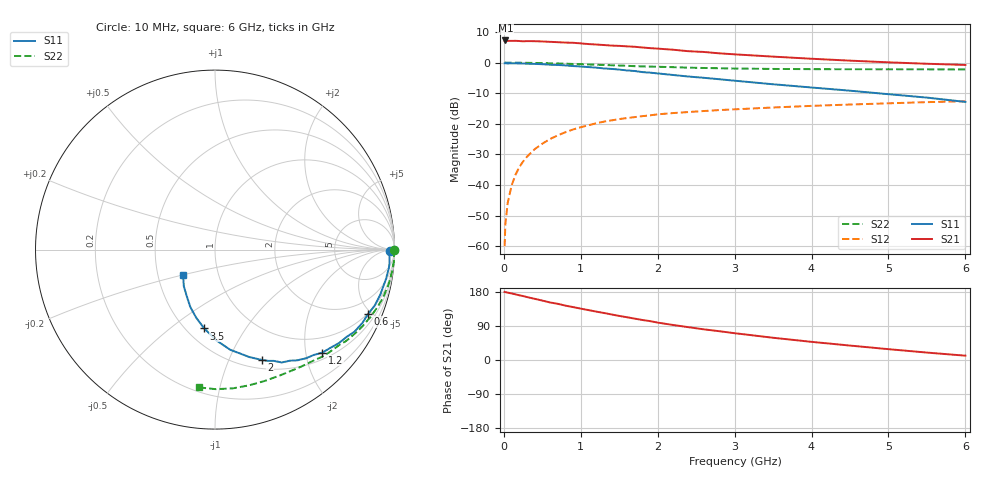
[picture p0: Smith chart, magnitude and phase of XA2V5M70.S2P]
! SIEMENS Discrete & RF Semiconductors
! BFY180
! Si NPN RF Bipolar Junction Transistor in MICRO-X
! VCE = 2.5 V  IC = 0.7 mA
! Common Emitter S-Parameters:  May  1997
# GHz  S  MA  R  50
!  f  S11  S21  S12  S22
! GHz  MAG  ANG  MAG  ANG  MAG  ANG  MAG  ANG
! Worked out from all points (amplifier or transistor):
!   36 points, 10 MHz to 6 GHz, reference 50 ohm
!   highest |S21| = 7.3 dB at 20 MHz (marker M1)
!   |S21| within 3 dB of that: start of sweep to 2.186 GHz
!   unconditionally stable (mu >= 1): 4.433 GHz to end of sweep
!   at 250 MHz: K = 0.07, MSG = 19.6 dB, |S12| = -32.3 dB
!   at 1.4 GHz: K = 0.44, MSG = 12.2 dB, |S12| = -18.9 dB
!   at 6 GHz: K = 1.05, MAG = 4.6 dB, |S12| = -12.6 dB
!   S11 on the Smith chart (normalised r, x): 10 MHz: 73, -14; 600 MHz: 0.96, -4.78; 1.2 GHz: 0.64, -2.34; 2 GHz: 0.60, -1.33; 3.5 GHz: 0.61, -0.67; 6 GHz: 0.67, -0.20
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0.01  0.9738 -0.3  2.251 179.8  0.001 84.4  0.9988 -0.1
0.02  0.9792 -0.9  2.305 179.1  0.0023 85.0  0.9999 -0.5
0.05  0.9717 -1.8  2.267 177.8  0.0051 88.1  0.9972 -1.2
0.1  0.9753 -4.0  2.267 175.7  0.0097 86.8  0.9977 -2.5
0.15  0.9745 -6.0  2.275 173.3  0.0146 87.3  0.9986 -3.7
0.2  0.9703 -7.7  2.258 170.9  0.0195 84.7  0.9965 -5.0
0.4  0.9541 -15.4  2.242 161.5  0.0384 79.2  0.9889 -9.8
0.6  0.9254 -22.8  2.189 151.9  0.0564 72.9  0.9773 -14.5
0.9  0.8798 -33.6  2.111 139.6  0.0808 65.0  0.9521 -21.3
1.1  0.8456 -40.2  2.013 131.7  0.0947 60.1  0.9338 -25.5
1.2  0.8291 -43.8  1.978 127.7  0.102 57.7  0.9255 -27.7
1.5  0.7699 -53.2  1.88 116.3  0.1194 51.5  0.8975 -33.4
1.7  0.7306 -59.4  1.818 109.2  0.1286 47.9  0.8755 -36.9
2  0.6669 -67.1  1.695 98.7  0.1429 43.0  0.8563 -41.9
2.2  0.6285 -72.3  1.627 92.4  0.1499 39.6  0.8432 -45.2
2.6  0.565 -81.3  1.495 80.9  0.1618 34.7  0.8179 -50.8
3  0.5068 -89.0  1.367 70.7  0.1724 30.0  0.8014 -56.4
3.5  0.4432 -97.8  1.255 58.7  0.1849 25.3  0.7891 -62.7
4  0.3925 -105.6  1.158 47.9  0.1965 20.8  0.7825 -69.2
4.5  0.3481 -113.3  1.078 38.1  0.2067 16.5  0.7796 -75.9
5.5  0.2683 -130.4  0.959 19.6  0.2261 8.2  0.7776 -89.7
6  0.2282 -140.9  0.917 11.4  0.234 3.8  0.773 -96.7
